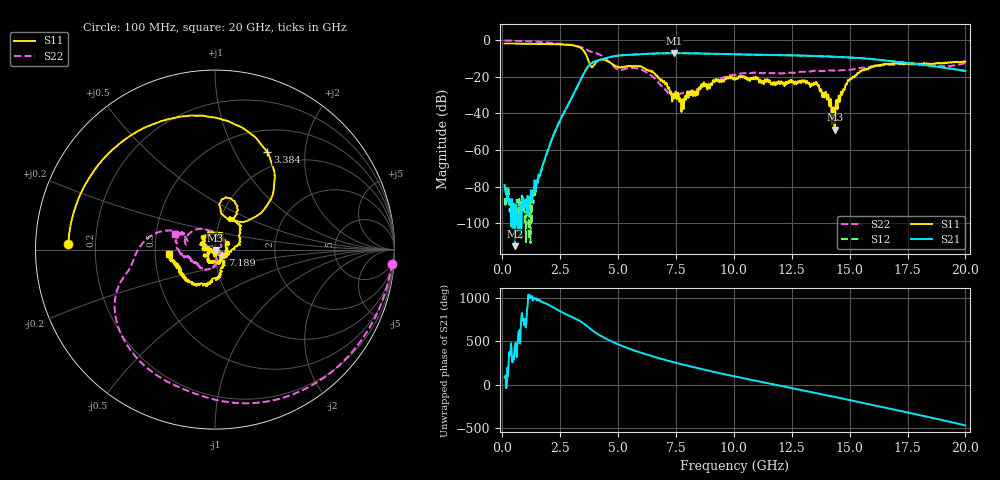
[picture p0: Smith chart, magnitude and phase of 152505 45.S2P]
!  2-Port S-parameters saved by WinCal
! VAR MeasName=S-Parameters (CALIBRATED_DATA) read from VNA (N5230C)
! VAR MeasDate=4/10/2015 9:33:01 AM
! VAR NAME=152505 45
! VAR FILENAME=152505 45.S2P
! VAR DATE=4/10/2015 9:33:01 AM
! VAR PHYS_PORTS=1,2
# Hz S DB R 50
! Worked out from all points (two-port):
!   801 points, 100 MHz to 20 GHz, reference 50 ohm
!   highest |S21| = -7.04 dB at 7.413 GHz (marker M1); lowest = -112.6 dB at 547.8 MHz (marker M2)
!   |S21| within 3 dB of the highest: 4.389 GHz to 15.73 GHz (11.35 GHz wide, 113 % of centre)
!   lowest |S11| = -48.9 dB at 14.35 GHz (marker M3), VSWR 1.01, Z = 50.3 - j0.21 ohm
!   |S11| at or under -10 dB: 3.69 GHz to end of sweep
!   |S22| runs from -30.8 to -0.1 dB; largest |S21 - S12| = 0.0065
!   S11 on the Smith chart (normalised r, x): 100 MHz: 0.10, +0.02; 3.384 GHz: 0.78, +1.36; 7.189 GHz: 1.08, -0.07; 20 GHz: 0.59, -0.03
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1e8  -1.75 177.6  -79.10 83.4  -86.30 3.5  -0.09 -4.6
5.4775e8  -1.77 167.0  -112.63 106.3  -96.28 153.4  -0.27 -22.4
1.418375e9  -1.90 145.3  -79.40 -94.6  -84.66 -71.2  -0.69 -57.6
2.463125e9  -2.20 113.4  -44.63 130.6  -44.66 130.8  -1.92 -100.9
3.3835e9  -4.21 61.7  -21.60 7.5  -21.60 7.8  -3.60 -147.4
3.43325e9  -4.68 57.7  -20.32 -0.8  -20.31 -0.5  -3.83 -150.3
3.856125e9  -14.76 61.8  -12.51 -89.1  -12.53 -88.9  -6.35 -168.2
4.478e9  -11.11 65.5  -9.72 170.0  -9.76 170.1  -10.12 160.8
5.22425e9  -14.67 65.1  -8.16 79.7  -8.16 79.9  -15.94 169.9
5.9705e9  -14.08 41.9  -7.64 9.3  -7.62 9.3  -15.85 139.0
6.741625e9  -20.91 -1.9  -7.16 -53.0  -7.16 -53.2  -23.08 77.1
7.189375e9  -25.65 -37.4  -7.09 -86.4  -7.10 -86.2  -28.99 15.3
7.41325e9  -30.00 -71.6  -7.04 -102.4  -7.05 -102.4  -30.05 -23.8
7.7615e9  -35.37 -148.2  -7.08 -126.6  -7.07 -126.4  -29.08 -66.7
8.60725e9  -24.00 172.3  -7.22 179.0  -7.21 178.7  -25.77 -79.3
1.005e10  -20.58 127.0  -7.61 94.0  -7.67 93.8  -18.85 -107.9
1.171662e10  -23.76 -7.1  -8.05 2.7  -8.07 2.6  -18.01 -141.3
1.338325e10  -24.18 -142.0  -8.58 -88.5  -8.53 -88.3  -16.78 -152.7
1.435338e10  -48.90 -35.6  -8.99 -142.2  -8.99 -142.0  -16.55 -163.8
1.5025e10  -20.93 -56.6  -9.45 -179.9  -9.45 -179.6  -16.06 -164.7
1.669162e10  -12.73 -122.6  -11.25 84.8  -11.17 84.1  -13.47 176.0
2e10  -11.70 -174.8  -16.82 -110.9  -16.83 -110.8  -12.36 158.9
